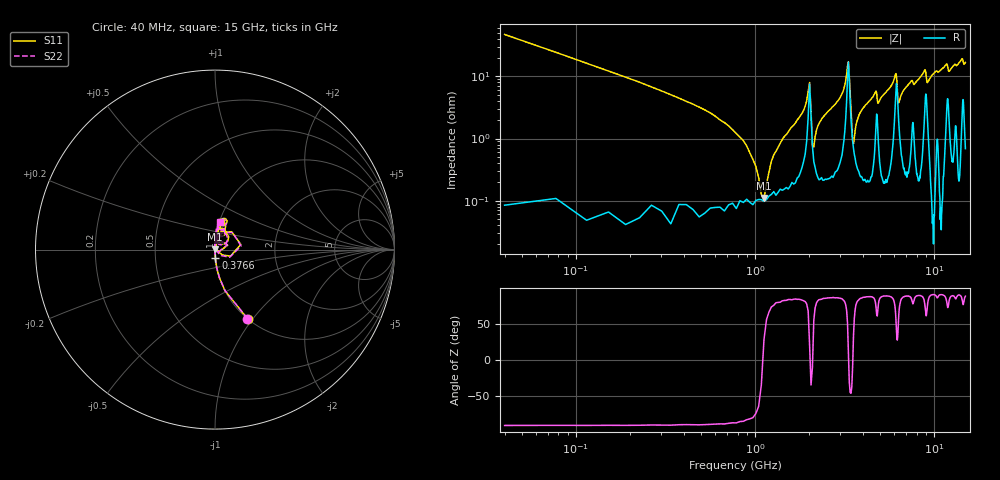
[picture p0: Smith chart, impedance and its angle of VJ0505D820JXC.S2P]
! VJ0505D820JXC
! MLCC placed on 25 mil thick microstrip substrate in series configuraton.
! DATE 06/29/2018  09:32
! CORRECTED  DATA
# GHz  S  MA  R  50.00
!  FREQ  S11M  S11A  S21M  S21A  S12M  S12A  S22M  S22A
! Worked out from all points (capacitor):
!   401 points, 40 MHz to 15 GHz, reference 50 ohm
!   read as one part in series: C = 84 pF near 114.8 MHz
!   lowest |Z| = 110 mohm at 1.125 GHz (marker M1)
!   series resonance near 1.109 GHz, so ESL is about 250 pH
!   S11 on the Smith chart (normalised r, x): 40 MHz: 1.00, -0.95; 376.6 MHz: 1.00, -0.09; 15 GHz: 1.02, +0.32
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0.04  0.4283 -64.7  0.9026 25.2  0.9039 25.3  0.4245 -64.8
0.3766  0.04451 -87.5  0.9971 2.5  0.9973 2.6  0.04441 -87.7
0.788  0.0111 -89.3  0.998 0.7  0.9984 0.8  0.01086 -92.0
0.9376  0.004686 -88.2  0.998 0.3  0.9981 0.5  0.004578 -92.2
1.0124  0.002501 -80.1  0.9979 0.2  0.9982 0.3  0.002448 -96.4
1.1246  0.001974 82.0  0.998 0.0  0.998 0.1  0.002142 100.1
1.3116  0.007514 86.4  0.9976 -0.3  0.9977 -0.2  0.007546 91.3
1.9474  0.04209 76.7  0.989 -2.1  0.9889 -2.1  0.04232 78.1
2.1718  0.01259 78.3  0.9953 -0.5  0.9952 -0.4  0.01287 82.3
2.5458  0.0297 86.1  0.9962 -1.4  0.9961 -1.3  0.03042 87.1
3.2938  0.1361 47.1  0.9074 -5.7  0.9076 -5.6  0.1365 44.2
3.3686  0.09377 -22.8  0.915 3.0  0.9151 3.1  0.09215 -27.6
3.4808  0.01488 -18.4  0.9858 0.8  0.9859 0.8  0.01133 -29.3
3.5556  0.01176 49.5  0.9919 -0.0  0.9918 0.0  0.009426 66.4
3.9296  0.03205 83.2  0.9958 -1.4  0.9962 -1.3  0.03177 89.0
5.0516  0.0497 84.0  0.9945 -2.3  0.9948 -2.2  0.04871 87.6
6.0988  0.1098 64.4  0.9538 -5.1  0.9545 -5.0  0.1046 63.3
6.3606  0.04483 58.6  0.9794 -1.5  0.9798 -1.4  0.03881 69.2
7.52  0.0894 77.4  0.9843 -4.5  0.9849 -4.5  0.08995 81.8
10.0258  0.1144 82.7  0.9909 -6.2  0.9917 -6.3  0.117 85.5
12.5316  0.1308 77.3  0.9849 -7.7  0.9852 -7.8  0.1337 83.6
15  0.1575 77.4  0.979 -9.9  0.9795 -9.9  0.1559 79.1
